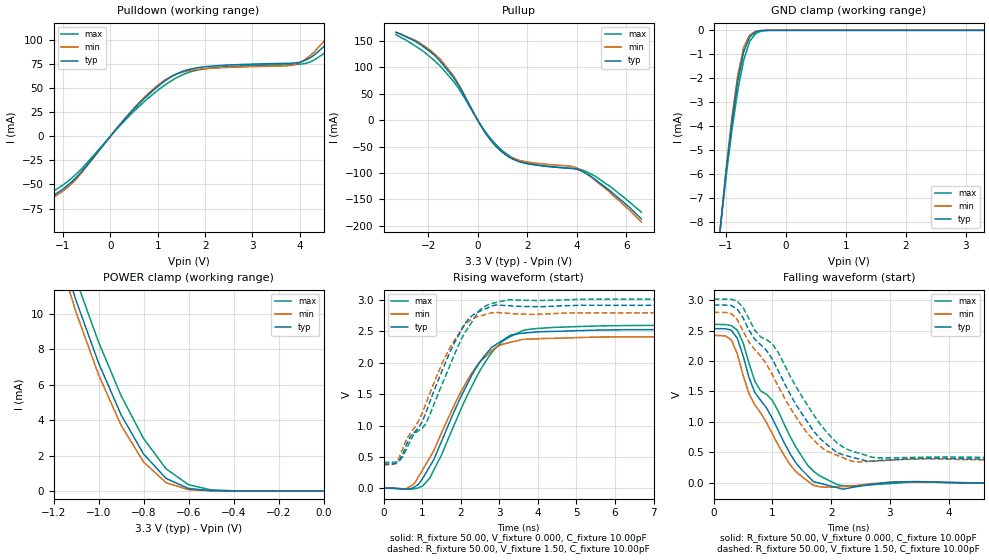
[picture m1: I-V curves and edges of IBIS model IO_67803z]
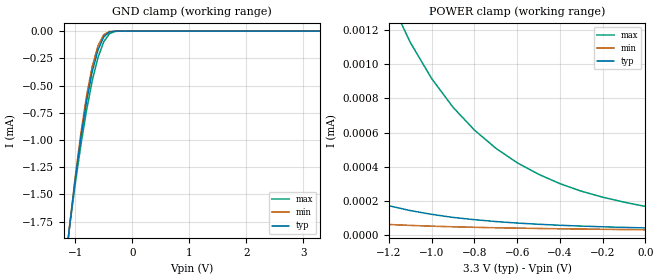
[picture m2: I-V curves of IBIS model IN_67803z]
| IBIS file 71v67803z.ibs created by s2ibis2 version 1.1
| North Carolina State University Electronics Research Laboratory  1995
[IBIS ver]   2.1
[File name]   71v67803z_pf.ibs
[File Rev]   1.1
[Date]   08/08/00
[Source]   Integrated Device Technology, Inc.
[Notes]   1. Temperatures: typ=25C, min=0C, max=70C 2. Cmos115_3v
   process. 3. Ramp rates based on 50 ohm load.
[Copyright]   Copyright 1998, Integrated Device Technology, Inc. Integrated
   Device Technology, Inc. ("IDT") hereby grants the user of this
   IBIS model a non-exclusive, nontransferable license to use
   this IBIS model under the following terms. The user is granted
   this license only to use the IBIS model and is not granted
   rights to sell, copy (except as needed to run the IBIS model),
   rent, lease or sub-license the IBIS model in whole or in part,
   or in modified form to anyone. The User may modify the IBIS
   model to suit its specific applications, but rights to
   derivative works and such modifications shall belong to IDT.
   This IBIS model is provided on an AS IS" basis and IDT makes
   absolutely no warranty with respect to the information
   contained herein. IDT DISCLAIMS AND CUSTOMER WAIVES ALL
   WARRANTIES, EXPRESS AND IMPLIED, INCLUDING WARRANTIES OF
   MERCHANTABILITY AND FITNESS FOR A PARTICULAR PURPOSE. THE
   ENTIRE RISK AS TO QUALITY AND PERFORMANCE IS WITH THE USER
   ACCORDINGLY, IN NO EVENT SHALL IDT BE LIABLE FOR ANY DIRECT OR
   INDIRECT DAMAGES, WHETHER IN CONTRACT OR TORT, INCLUDING ANY
   LOST PROFITS OR OTHER INCIDENTAL, CONSEQUENTIAL, EXEMPLARY, OR
   PUNITIVE DAMAGES ARISING OUT OF THE USE OR APPLICATION OF THE
   IBIS model. Further, IDT reserves the right to make changes
   without notice to any product herein to improve reliability,
   function, or design. IDT does not convey any license under
   patent rights or any other intellectual property rights,
   including those of third parties. IDT is not obligated to
   provide maintenance or support for the licensed IBIS model.
|   Component 71v67803z
[Component]   idt71v67803z
[Manufacturer]   Integrated Device Technology
|  This component uses the 100 pin TQFP pagage (PF)
[Package]
| variable   typ   min   max
R_pkg   4.77m   4.29m   5.25m
L_pkg   6.95nH   6.25nH   7.64nH
C_pkg   0.87pF   0.78pF   0.96pF
[Pin]  signal_name   model_name   R_pin   L_pin   C_pin
1   IOP3   IO_67803z
2   IO16   IO_67803z
3   IO17   IO_67803z
4   VDDQ   POWER
5   GND   GND
6   IO18   IO_67803z
7   IO19   IO_67803z
8   IO20   IO_67803z
9   IO21   IO_67803z
10   GND   GND
11   VDDQ   POWER
12   IO22   IO_67803z
13   IO23   IO_67803z
14   NFT   IN_67803z
15   VDD   POWER
16   NC   NC
17   GND   GND
18   IO24   IO_67803z
19   IO25   IO_67803z
20   VDDQ   POWER
21   GND   GND
22   IO26   IO_67803z
23   IO27   IO_67803z
24   IO28   IO_67803z
25   IO29   IO_67803z
26   GND   GND
27   VDDQ   POWER
28   IO30   IO_67803z
29   IO31   IO_67803z
30   IOP4   IO_67803z
31   NLBO   IN_67803z
32   A5   IN_67803z
33   A4   IN_67803z
34   A3   IN_67803z
35   A2   IN_67803z
36   A1   IN_67803z
37   A0   IN_67803z
38   NC   NC
39   NC   NC
40   GND   GND
41   VDD   POWER
42   NC   NC
43   A17   IN_67803z
44   A10   IN_67803z
45   A11   IN_67803z
46   A12   IN_67803z
47   A13   IN_67803z
48   A14   IN_67803z
49   A15   IN_67803z
50   A16   IN_67803z
51   IOP1   IO_67803z
52   IO0   IO_67803z
53   IO1   IO_67803z
54   VDDQ   POWER
55   GND   GND
56   IO2   IO_67803z
57   IO3   IO_67803z
58   IO4   IO_67803z
59   IO5   IO_67803z
60   GND   GND
61   VDDQ   POWER
62   IO6   IO_67803z
63   IO7   IO_67803z
64   ZZ   IN_67803z
65   VDD   POWER
66   NC   NC
67   GND   GND
68   IO8   IO_67803z
69   IO9   IO_67803z
70   VDDQ   POWER
71   GND   GND
72   IO10   IO_67803z
73   IO11   IO_67803z
74   IO12   IO_67803z
75   IO13   IO_67803z
76   GND   GND
77   VDDQ   POWER
78   IO14   IO_67803z
79   IO15   IO_67803z
80   IOP2   IO_67803z
81   A9   IN_67803z
82   A8   IN_67803z
83   NADV   IN_67803z
84   NADSP   IN_67803z
85   NADSC   IN_67803z
86   NOE   IN_67803z
87   NBWE   IN_67803z
88   NGW   IN_67803z
89   CLK   IN_67803z
90   GND   GND
91   VDD   POWER
92   NCS1   IN_67803z
93   NBW1   IN_67803z
94   NBW2   IN_67803z
95   NBW3   IN_67803z
96   NBW4   IN_67803z
97   CS0   IN_67803z
98   NCE   IN_67803z
99   A7   IN_67803z
100   A6   IN_67803z
|NDAIN NDAIN   dummy_model
|OC   OC   dummy_model
|PUD   PUD   dummy_model
[Pin Mapping]  pulldown_ref   pullup_ref   gnd_clamp_ref   power_clamp_ref
1   EXTGND   EXTVDDQ   EXTGND   EXTVDD
2   EXTGND   EXTVDDQ   EXTGND   EXTVDD
3   EXTGND   EXTVDDQ   EXTGND   EXTVDD
4   NC   EXTVDDQ
5   EXTGND   NC
6   EXTGND   EXTVDDQ   EXTGND   EXTVDD
7   EXTGND   EXTVDDQ   EXTGND   EXTVDD
8   EXTGND   EXTVDDQ   EXTGND   EXTVDD
9   EXTGND   EXTVDDQ   EXTGND   EXTVDD
10   EXTGND   NC
11   NC   EXTVDDQ
12   EXTGND   EXTVDDQ   EXTGND   EXTVDD
13   EXTGND   EXTVDDQ   EXTGND   EXTVDD
14   EXTGND   EXTVDDQ   EXTGND   EXTVDD
15   NC   EXTVDD
16   NC   NC   NC   NC
17   EXTGND   NC
18   EXTGND   EXTVDDQ   EXTGND   EXTVDD
19   EXTGND   EXTVDDQ   EXTGND   EXTVDD
20   NC   EXTVDDQ
21   EXTGND   NC
22   EXTGND   EXTVDDQ   EXTGND   EXTVDD
23   EXTGND   EXTVDDQ   EXTGND   EXTVDD
24   EXTGND   EXTVDDQ   EXTGND   EXTVDD
25   EXTGND   EXTVDDQ   EXTGND   EXTVDD
26   EXTGND   NC
27   NC   EXTVDDQ
28   EXTGND   EXTVDDQ   EXTGND   EXTVDD
29   EXTGND   EXTVDDQ   EXTGND   EXTVDD
30   EXTGND   EXTVDDQ   EXTGND   EXTVDD
31   EXTGND   EXTVDDQ   EXTGND   EXTVDD
32   EXTGND   EXTVDDQ   EXTGND   EXTVDD
33   EXTGND   EXTVDDQ   EXTGND   EXTVDD
34   EXTGND   EXTVDDQ   EXTGND   EXTVDD
35   EXTGND   EXTVDDQ   EXTGND   EXTVDD
36   EXTGND   EXTVDDQ   EXTGND   EXTVDD
37   EXTGND   EXTVDDQ   EXTGND   EXTVDD
38   NC   NC   NC   NC
39   NC   NC   NC   NC
40   EXTGND   NC
41   NC   EXTVDD
42   NC   NC   NC   NC
43   EXTGND   EXTVDDQ   EXTGND   EXTVDD
44   EXTGND   EXTVDDQ   EXTGND   EXTVDD
45   EXTGND   EXTVDDQ   EXTGND   EXTVDD
46   EXTGND   EXTVDDQ   EXTGND   EXTVDD
47   EXTGND   EXTVDDQ   EXTGND   EXTVDD
48   EXTGND   EXTVDDQ   EXTGND   EXTVDD
49   EXTGND   EXTVDDQ   EXTGND   EXTVDD
50   EXTGND   EXTVDDQ   EXTGND   EXTVDD
51   EXTGND   EXTVDDQ   EXTGND   EXTVDD
52   EXTGND   EXTVDDQ   EXTGND   EXTVDD
53   EXTGND   EXTVDDQ   EXTGND   EXTVDD
54   NC   EXTVDDQ
55   EXTGND   NC
56   EXTGND   EXTVDDQ   EXTGND   EXTVDD
57   EXTGND   EXTVDDQ   EXTGND   EXTVDD
58   EXTGND   EXTVDDQ   EXTGND   EXTVDD
59   EXTGND   EXTVDDQ   EXTGND   EXTVDD
60   EXTGND   NC
61   NC   EXTVDDQ
62   EXTGND   EXTVDDQ   EXTGND   EXTVDD
63   EXTGND   EXTVDDQ   EXTGND   EXTVDD
64   EXTGND   EXTVDDQ   EXTGND   EXTVDD
65   NC   EXTVDD
66   NC   NC   NC   NC
67   EXTGND   NC
68   EXTGND   EXTVDDQ   EXTGND   EXTVDD
69   EXTGND   EXTVDDQ   EXTGND   EXTVDD
70   NC   EXTVDDQ
71   EXTGND   NC
72   EXTGND   EXTVDDQ   EXTGND   EXTVDD
73   EXTGND   EXTVDDQ   EXTGND   EXTVDD
74   EXTGND   EXTVDDQ   EXTGND   EXTVDD
75   EXTGND   EXTVDDQ   EXTGND   EXTVDD
76   EXTGND   NC
77   NC   EXTVDDQ
78   EXTGND   EXTVDDQ   EXTGND   EXTVDD
79   EXTGND   EXTVDDQ   EXTGND   EXTVDD
80   EXTGND   EXTVDDQ   EXTGND   EXTVDD
81   EXTGND   EXTVDDQ   EXTGND   EXTVDD
82   EXTGND   EXTVDDQ   EXTGND   EXTVDD
83   EXTGND   EXTVDDQ   EXTGND   EXTVDD
84   EXTGND   EXTVDDQ   EXTGND   EXTVDD
85   EXTGND   EXTVDDQ   EXTGND   EXTVDD
86   EXTGND   EXTVDDQ   EXTGND   EXTVDD
87   EXTGND   EXTVDDQ   EXTGND   EXTVDD
88   EXTGND   EXTVDDQ   EXTGND   EXTVDD
89   EXTGND   EXTVDDQ   EXTGND   EXTVDD
90   EXTGND   NC
91   NC   EXTVDD
92   EXTGND   EXTVDDQ   EXTGND   EXTVDD
93   EXTGND   EXTVDDQ   EXTGND   EXTVDD
94   EXTGND   EXTVDDQ   EXTGND   EXTVDD
95   EXTGND   EXTVDDQ   EXTGND   EXTVDD
96   EXTGND   EXTVDDQ   EXTGND   EXTVDD
97   EXTGND   EXTVDDQ   EXTGND   EXTVDD
98   EXTGND   EXTVDDQ   EXTGND   EXTVDD
99   EXTGND   EXTVDDQ   EXTGND   EXTVDD
100   EXTGND   EXTVDDQ   EXTGND   EXTVDD
| Models and submodels in the file (2): IO_67803z (I/O), IN_67803z (Input)
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|NDAIN   NC   NC   NC   NC
|OC   NC   NC   NC   NC
|PUD   NC   NC   NC   NC
|   Model IO_67803z
[Model]   IO_67803z
Model_type   I/O
Polarity   Non-Inverting
Enable   Active-Low
Vinl =  0.800V
Vinh =  2.000V
Vmeas =  1.500V
Vref = 1.50   | AC test load as shown
Rref = 50.00   | in the datasheet
Cref = 0.00
C_comp   4.50pF   NA   NA
[Temperature Range]   25.00   0.000   70.00
[Pullup Reference]   3.30V   3.13V   3.46V
[Pulldown Reference]   0.000V   0.000V   0.000V
[POWER Clamp Reference]   3.30V   3.13V   3.46V
[GND Clamp Reference]   0.000V   0.000V   0.000V
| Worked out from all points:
|   slope of the pulldown table from 0 to 0.495 V, typ, clamps not added: 17.6 ohm
|   slope of the pullup table from 0 to 0.495 V, typ, clamps not added: 13.9 ohm
|   GND clamp passes 1 mA (typ) near -0.71 V on its own axis
|   POWER clamp passes 1 mA (typ) near -0.72 V on its own axis
|   rising waveform, R_fixture 50.00, V_fixture 0.000, C_fixture 10.00pF: 20-80 % time 1.17ns typ, 1.2ns min, 1.21ns max; typ from 0 V to 2.53 V
|   rising waveform, R_fixture 50.00, V_fixture 1.50, C_fixture 10.00pF: 20-80 % time 1.12ns typ, 1.12ns min, 1.18ns max; typ from 0.386 V to 2.92 V
|   falling waveform, R_fixture 50.00, V_fixture 0.000, C_fixture 10.00pF: 20-80 % time 767ps typ, 727ps min, 877ps max; typ from 2.53 V to 0 V
|   falling waveform, R_fixture 50.00, V_fixture 1.50, C_fixture 10.00pF: 20-80 % time 1.01ns typ, 962ps min, 1.13ns max; typ from 2.92 V to 0.386 V
[Pulldown]
| voltage   I(typ)   I(min)   I(max)
-3.3V     -94.34mA   -91.7mA    -94.53mA
-1.9V     -80.79mA   -81.69mA   -76.75mA
-1V       -54.82mA   -56.9mA    -50.58mA
700mV     38.31mA    39.55mA    35.26mA
1.5V      66.97mA    66.34mA    63.35mA
2.2V      73.13mA    70.87mA    71.3mA
3.9V      76.15mA    74.53mA    74.65mA
4.3V      84.18mA    87.33mA    79.08mA
4.7V      104mA      111mA      94.54mA
4.9V      117mA      127mA      106mA
5.1V      133mA      145mA      119mA
6.6V      326mA      353mA      291mA
[Pullup]
| voltage   I(typ)   I(min)   I(max)
-3.3V     167mA      166mA      162mA
-2.5V     149mA      151mA      140mA
-1.5V     111mA      115mA      102mA
-900mV    75.38mA    78.28mA    68.71mA
300mV     -22.92mA   -23.43mA   -21.2mA
700mV     -47.18mA   -47.54mA   -44.22mA
1.1V      -64.55mA   -63.95mA   -61.46mA
1.5V      -75.52mA   -73.42mA   -73.2mA
2V        -82.3mA    -78.91mA   -81.17mA
4V        -92.8mA    -90.45mA   -91.84mA
4.9V      -118mA     -120mA     -111mA
6.6V      -187mA     -193mA     -174mA
[GND_clamp]
| voltage   I(typ)   I(min)   I(max)
-3.3V     -86.36mA   -90mA      -80.77mA
-1.1V     -8.465mA   -8.484mA   -8.443mA
-1V       -6.026mA   -5.913mA   -6.205mA
-900mV    -3.877mA   -3.668mA   -4.205mA
-800mV    -2.116mA   -1.871mA   -2.51mA
-700mV    -884uA     -699uA     -1.223mA
-600mV    -270uA     -190uA     -451uA
-500mV    -63.71uA   -37.8uA    -131uA
-400mV    -8.97uA    -4.018uA   -27.41uA
-300mV    -726nA     -237nA     -3.489uA
3.3V      43.71nA    35.33nA    138nA
[POWER_clamp]
| voltage   I(typ)   I(min)   I(max)
-3.3V     168mA      174mA      158mA
-1.2V     14.83mA    14.24mA    15.91mA
-1.1V     10.76mA    10.1mA     11.94mA
-1V       7.233mA    6.571mA    8.412mA
-900mV    4.308mA    3.713mA    5.391mA
-800mV    2.09mA     1.639mA    2.962mA
-700mV    706uA      466uA      1.252mA
-600mV    138uA      71.27uA    348uA
-500mV    16.75uA    6.941uA    60.62uA
-400mV    1.562uA    511nA      8.096uA
0V        43.71nA    32.91nA    169nA
[Ramp]
| variable   typ   min   max
dV/dt_r   1.52/0.81n   1.45/0.83n   1.56/0.81n
dV/dt_f   1.43/0.68n   1.38/0.69n   1.46/0.71n
R_load = 50.00
[Rising Waveform]
R_fixture = 50.00
V_fixture = 0.000
C_fixture = 10.00pF
R_dut = 4.77m
L_dut = 6.95nH
C_dut = 8.66pF
| time   V(typ)   V(min)   V(max)
0s        0V         0V         0V
700ps     -7.227mV   34.29mV    -13.98mV
900ps     59.78mV    179mV      5.183mV
1.2ns     353mV      490mV      168mV
1.9ns     1.322V     1.415V     1.113V
2.3ns     1.819V     1.85V      1.644V
2.8ns     2.247V     2.195V     2.163V
3.3ns     2.443V     2.329V     2.421V
4.4ns     2.501V     2.391V     2.565V
9.9ns     2.531V     2.418V     2.6V
[Rising Waveform]
R_fixture = 50.00
V_fixture = 1.50
C_fixture = 10.00pF
R_dut = 4.77m
L_dut = 6.95nH
C_dut = 8.66pF
| time   V(typ)   V(min)   V(max)
0s        386mV      375mV      412mV
400ps     430mV      484mV      431mV
600ps     710mV      790mV      637mV
800ps     894mV      966mV      878mV
1.1ns     1.214V     1.357V     1.037V
1.6ns     2.001V     2.1V       1.782V
2.1ns     2.621V     2.607V     2.476V
2.5ns     2.825V     2.747V     2.849V
2.8ns     2.905V     2.797V     2.945V
9.9ns     2.919V     2.798V     3.017V
[Falling Waveform]
R_fixture = 50.00
V_fixture = 0.000
C_fixture = 10.00pF
R_dut = 4.77m
L_dut = 6.95nH
C_dut = 8.66pF
| time   V(typ)   V(min)   V(max)
0s        2.531V     2.418V     2.6V
300ps     2.505V     2.346V     2.579V
400ps     2.373V     2.12V      2.507V
600ps     1.729V     1.461V     1.964V
700ps     1.483V     1.279V     1.666V
1ns       1.053V     799mV      1.349V
1.3ns     477mV      297mV      760mV
1.7ns     18.16mV    -43.07mV   189mV
2.3ns     -88.4mV    -58.31mV   -53.25mV
9.9ns     -460nV     350nV      -2.864uV
[Falling Waveform]
R_fixture = 50.00
V_fixture = 1.50
C_fixture = 10.00pF
R_dut = 4.77m
L_dut = 6.95nH
C_dut = 8.66pF
| time   V(typ)   V(min)   V(max)
0s        2.919V     2.798V     3.017V
300ps     2.91V      2.777V     3.013V
500ps     2.705V     2.489V     2.877V
700ps     2.354V     2.185V     2.504V
1.1ns     1.837V     1.582V     2.135V
1.6ns     992mV      806mV      1.269V
1.9ns     649mV      529mV      859mV
2.2ns     458mV      411mV      588mV
2.8ns     364mV      359mV      408mV
9.9ns     386mV      375mV      412mV
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|   Model IN_67803z
[Model]   IN_67803z
Model_type   Input
Vinl =  0.800V
Vinh =  2.000V
Vmeas =  1.500V
C_comp   4.50pF   NA   NA
[Temperature Range]   25.00   0.000   70.00
[Pullup Reference]   3.30V   3.13V   3.46V
[Pulldown Reference]   0.000V   0.000V   0.000V
[POWER Clamp Reference]   3.30V   3.13V   3.46V
[GND Clamp Reference]   0.000V   0.000V   0.000V
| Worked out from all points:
|   GND clamp passes 1 mA (typ) near -0.91 V on its own axis
[GND_clamp]
| voltage   I(typ)   I(min)   I(max)
-3.3V     -19.19mA   -20.68mA   -17.2mA
-1.2V     -2.269mA   -2.302mA   -2.234mA
-1.1V     -1.796mA   -1.797mA   -1.803mA
-1V       -1.363mA   -1.34mA    -1.405mA
-900mV    -976uA     -935uA     -1.043mA
-800mV    -641uA     -591uA     -723uA
-700mV    -369uA     -320uA     -451uA
-600mV    -172uA     -134uA     -241uA
-500mV    -53.18uA   -33.05uA   -98.11uA
-400mV    -8.241uA   -3.78uA    -23.91uA
-200mV    -38.37nA   -10.49nA   -284nA
3.3V      43.77nA    35.15nA    138nA
[POWER_clamp]
| voltage   I(typ)   I(min)   I(max)
-3.3V     17.79uA    4.255uA    102uA
-2.8V     6.037uA    1.322uA    40.55uA
-2.4V     2.434uA    516nA      18.29uA
-2.1V     1.214uA    264nA      9.776uA
-1.9V     764nA      176nA      6.367uA
-1.7V     485nA      122nA      4.123uA
-1.2V     173nA      63.69nA    1.392uA
-1.1V     145nA      58.36nA    1.127uA
-900mV    105nA      50.32nA    748nA
-700mV    80.85nA    44.61nA    509nA
-400mV    59.15nA    38.69nA    302nA
0V        43.77nA    32.91nA    169nA
